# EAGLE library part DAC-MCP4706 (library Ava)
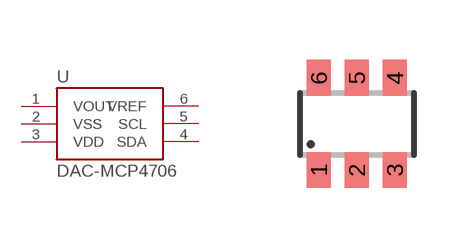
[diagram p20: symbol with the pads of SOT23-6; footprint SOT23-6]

Designator prefix -

## DAC-MCP4706  [SOT23-6]
1  VOUT
2  VSS
3  VDD
4  SDA
5  SCL
6  VREF

## Footprint SOT23-6 (pad centres in mm)
smd 0.6 x 0.9: 1 -0.95,-1.15; 2 0,-1.15; 3 0.95,-1.15; 4 0.95,1.15; 5 0,1.15; 6 -0.95,1.15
